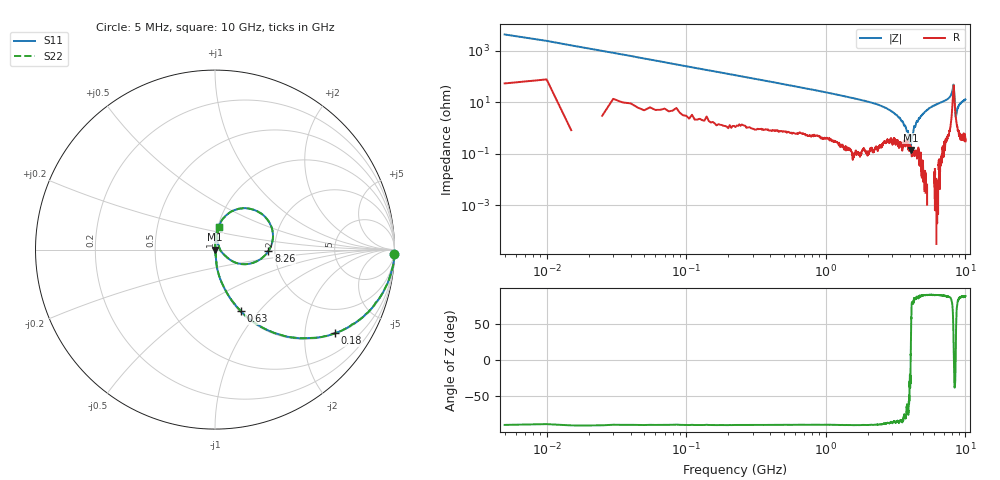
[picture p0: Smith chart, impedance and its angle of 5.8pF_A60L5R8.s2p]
! Amotech Co.,Ltd.
! http://www.amotech.co.kr/
! Part Number: A60L5R8
! These Parameters are Measured in Series Mode Connection
! Operation Temp=25[degC], DC Bias Voltage=0[V]
! Freq. Start=5[MHz] Stop=10[GHz], 2000[Steps]
! Date: Monday, July 14, 2020, 09:32:41
# GHZ S RI R 50.000000
!Freq.(Hz) S11(Real) S11(Imag) S21(Real) S21(Imag) S12(Real) S12(Imag) S22(Real) S22(Imag)
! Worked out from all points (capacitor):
!   2000 points, 5 MHz to 10 GHz, reference 50 ohm
!   read as one part in series: C = 6.25 pF near 55 MHz
!   lowest |Z| = 141 mohm at 4.05 GHz (marker M1)
!   series resonance near 4.051 GHz, so ESL is about 250 pH
!   S11 on the Smith chart (normalised r, x): 5 MHz: 2, -88; 180 MHz: 1.03, -2.85; 630 MHz: 1.01, -0.80; 8.26 GHz: 1.85, -0.03; 10 GHz: 1.01, +0.26
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0.005  0.9992 -0.0228  0.000803 0.0228  0.000803 0.0228  0.9992 -0.0228
0.08  0.9062 -0.2841  0.0938 0.2841  0.0938 0.2841  0.9062 -0.2841
0.18  0.6687 -0.4661  0.3313 0.4661  0.3313 0.4661  0.6687 -0.4661
0.375  0.3194 -0.4599  0.6806 0.4599  0.6806 0.4599  0.3194 -0.4599
0.63  0.1421 -0.3419  0.8579 0.3419  0.8579 0.3419  0.1421 -0.3419
1.675  0.0187 -0.1315  0.9813 0.1315  0.9813 0.1315  0.0187 -0.1315
2.7  0.00622 -0.0598  0.9938 0.0598  0.9938 0.0598  0.00622 -0.0598
3.34  0.00276 -0.0253  0.9972 0.0253  0.9972 0.0253  0.00276 -0.0253
3.855  0.00283 -0.00717  0.9972 0.00717  0.9972 0.00717  0.00283 -0.00717
4.005  0.0021 -0.000753  0.9979 0.000753  0.9979 0.000753  0.0021 -0.000753
4.05  0.0014 -9.66e-05  0.9986 9.66e-05  0.9986 9.66e-05  0.0014 -9.66e-05
4.31  0.00095 0.0116  0.9991 -0.0116  0.9991 -0.0116  0.00095 0.0116
5.005  0.00144 0.0369  0.9986 -0.0369  0.9986 -0.0369  0.00144 0.0369
6.67  0.0103 0.0978  0.9897 -0.0978  0.9897 -0.0978  0.0103 0.0978
7.675  0.0299 0.1484  0.9701 -0.1484  0.9701 -0.1484  0.0299 0.1484
8.105  0.1549 0.2307  0.8451 -0.2307  0.8451 -0.2307  0.1549 0.2307
8.26  0.2974 -0.00835  0.7026 0.00835  0.7026 0.00835  0.2974 -0.00835
8.335  0.1488 -0.0808  0.8512 0.0808  0.8512 0.0808  0.1488 -0.0808
8.49  0.0342 -0.0102  0.9658 0.0102  0.9658 0.0102  0.0342 -0.0102
8.55  0.024 0.012  0.976 -0.012  0.976 -0.012  0.024 0.012
8.965  0.0117 0.0743  0.9883 -0.0743  0.9883 -0.0743  0.0117 0.0743
10  0.0195 0.1271  0.9805 -0.1271  0.9805 -0.1271  0.0195 0.1271
